(* Logix 5000 AddOnInstructionDefinition export POINT_ENC; software revision 30.00 *)

TYPE POINT :   // A point on an Edwards-curve represented in extended homogeneous coordinates
STRUCT
   X : DINT[22];
   Y : DINT[22];
   Z : DINT[22];
   T : DINT[22];
END_STRUCT
END_TYPE

ADD_ON_INSTRUCTION D_SHR   (* revision 1.0 20170524, vendor Kenneth A. Fischer *)
// DINT bit shift right of the 32-bit argument Inp_A by Inp_B bits with paddding by zeros on the right
// Revision note:
// Rev1.0: 20170524 - Initial Release
VAR_IN_OUT
   Inp_A : DINT; {required}   // 64-bit Integer to be right circular rotated
END_VAR
VAR_INPUT
   Inp_B : INT; {required}   // Number of bits to shift
END_VAR
VAR_IN_OUT
   Out : DINT; {required}   // Result
END_VAR
VAR
   BSR_Cntrl : CONTROL := (LEN := 32);
   ONS : BOOL;
   Source_Bit : BOOL;
   Wrk_InpA : DINT[2];
END_VAR

ROUTINE Logic   (* ladder *)
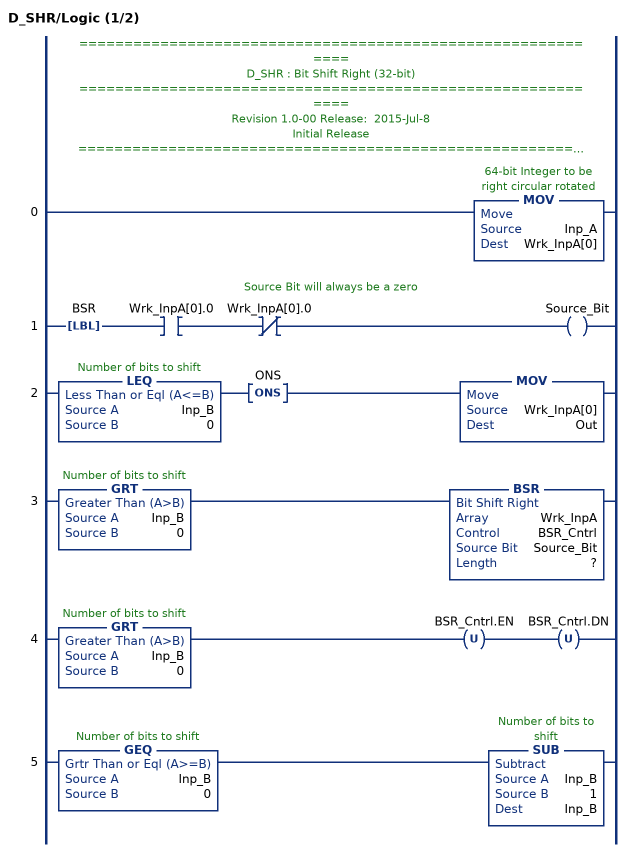
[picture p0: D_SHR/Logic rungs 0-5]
   // ============================================================
   // D_SHR : Bit Shift Right (32-bit)
   // ============================================================
   // Revision 1.0-00 Release:  2015-Jul-8
   // Initial Release
   // ============================================================
   // Performs a right bit shift of the 32-bit argument Inp_A by the
   // number of bits defined in the 16-bit argument Inp_B, with padding by zeros.
   0: MOV(Inp_A,Wrk_InpA[0]);
   // Source Bit will always be a zero
   1: LBL(BSR)XIC(Wrk_InpA[0].0)XIO(Wrk_InpA[0].0)OTE(Source_Bit);
   2: LEQ(Inp_B,0)ONS(ONS)MOV(Wrk_InpA[0],Out);
   3: GRT(Inp_B,0)BSR(Wrk_InpA,BSR_Cntrl,Source_Bit,?);
   4: GRT(Inp_B,0)OTU(BSR_Cntrl.EN)OTU(BSR_Cntrl.DN);
   5: GEQ(Inp_B,0)SUB(Inp_B,1,Inp_B);
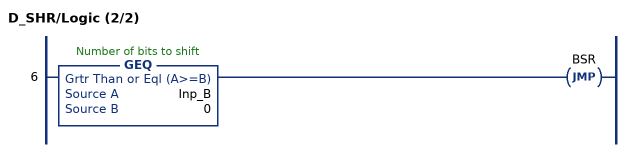
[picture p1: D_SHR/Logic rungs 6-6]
   6: GEQ(Inp_B,0)JMP(BSR);
END_ROUTINE
END_ADD_ON_INSTRUCTION

ADD_ON_INSTRUCTION B256_NRED   (* revision 1.0 20170916, vendor Kenneth A. Fischer *)
// Reduce 256-bit integer stored in 22 pieces by propagating carries
// Revision note:
// Rev1.0: 20170916 - Initial Release
VAR_IN_OUT
   Inp_C : DINT[22]; {required}
END_VAR
VAR
   D_SHR : D_SHR;
   temp : DINT;
   i : INT;
END_VAR

ROUTINE Logic   (* ladder *)
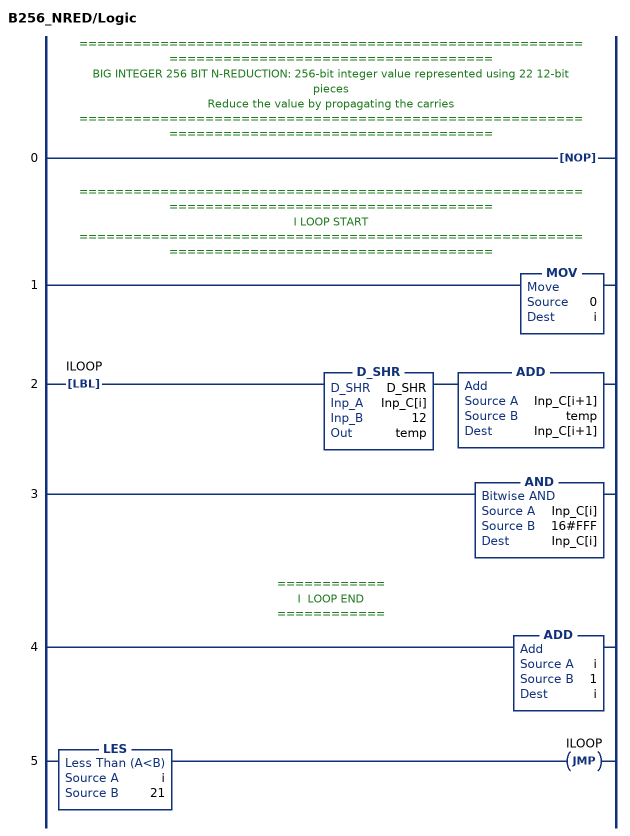
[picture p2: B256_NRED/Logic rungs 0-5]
   // ============================================================================================
   // BIG INTEGER 256 BIT N-REDUCTION: 256-bit integer value represented using 22 12-bit pieces
   // Reduce the value by propagating the carries
   // ============================================================================================
   0: NOP();
   // ============================================================================================
   // I LOOP START
   // ============================================================================================
   1: MOV(0,i);
   2: LBL(ILOOP)D_SHR(D_SHR,Inp_C[i],12,temp)ADD(Inp_C[i+1],temp,Inp_C[i+1]);
   3: AND(Inp_C[i],16#FFF,Inp_C[i]);
   // ============
   // I  LOOP END
   // ============
   4: ADD(i,1,i);
   5: LES(i,21)JMP(ILOOP);
END_ROUTINE
END_ADD_ON_INSTRUCTION

ADD_ON_INSTRUCTION B256_FRED   (* revision 1.0 20170916, vendor Kenneth A. Fischer *)
// fast_reduce:  reduce by propagating the carries starting at a particular offset and stoping once the carry becomes zero
// Revision note:
// Rev1.0: 20170916 - Initial Release
VAR_IN_OUT
   Inp_C : DINT[22]; {required}
END_VAR
VAR_INPUT
   Inp_offset : INT; {required}
END_VAR
VAR
   i : INT;
   carry : DINT;
   D_SHR : D_SHR;
END_VAR

ROUTINE Logic   (* ladder *)
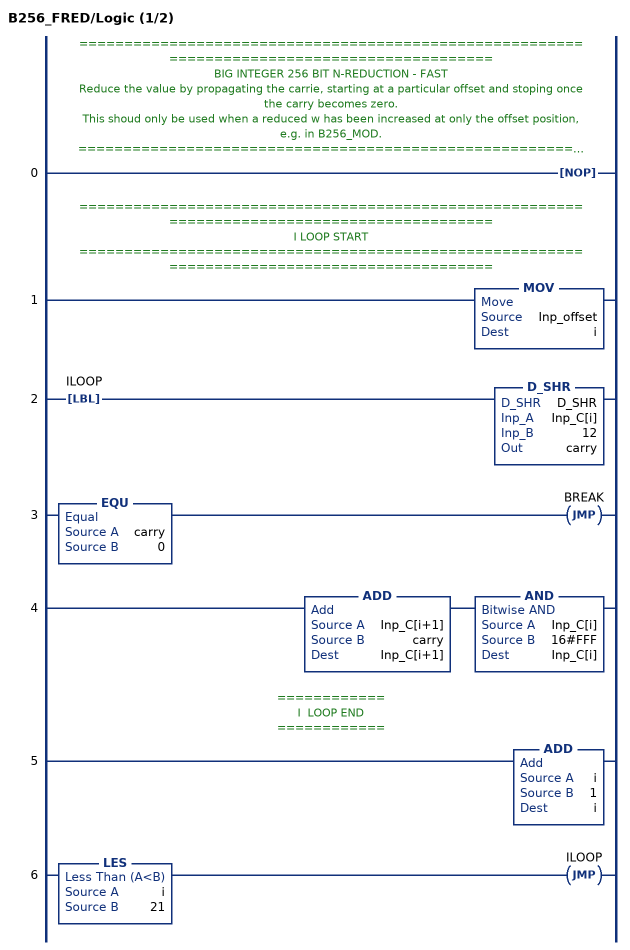
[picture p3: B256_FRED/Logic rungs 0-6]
   // ============================================================================================
   // BIG INTEGER 256 BIT N-REDUCTION - FAST
   // Reduce the value by propagating the carrie, starting at a particular offset and stoping once the carry becomes zero.
   // This shoud only be used when a reduced w has been increased at only the offset position, e.g. in B256_MOD.
   // ============================================================================================
   0: NOP();
   // ============================================================================================
   // I LOOP START
   // ============================================================================================
   1: MOV(Inp_offset,i);
   2: LBL(ILOOP)D_SHR(D_SHR,Inp_C[i],12,carry);
   3: EQU(carry,0)JMP(BREAK);
   4: ADD(Inp_C[i+1],carry,Inp_C[i+1])AND(Inp_C[i],16#FFF,Inp_C[i]);
   // ============
   // I  LOOP END
   // ============
   5: ADD(i,1,i);
   6: LES(i,21)JMP(ILOOP);
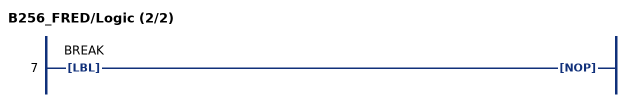
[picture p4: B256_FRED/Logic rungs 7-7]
   7: LBL(BREAK)NOP();
END_ROUTINE
END_ADD_ON_INSTRUCTION

ADD_ON_INSTRUCTION D_SHL   (* revision 1.0 20170524, vendor Kenneth A. Fischer *)
// DINT bit shift left of the 32-bit argument Inp_A by Inp_B bits with paddding by zeros on the right
// Revision note:
// Rev1.0: 20170524 - Initial Release
VAR_IN_OUT
   Inp_A : DINT; {required}   // 64-bit Integer to be right circular rotated
END_VAR
VAR_INPUT
   Inp_B : INT; {required}   // Number of bits to shift
END_VAR
VAR_IN_OUT
   Out : DINT; {required}   // Result
END_VAR
VAR
   Wrk_InpA : DINT[2];
   Source_Bit : BOOL;
   ONS : BOOL;
   BSL_Cntrl : CONTROL := (LEN := 32);
END_VAR

ROUTINE Logic   (* ladder *)
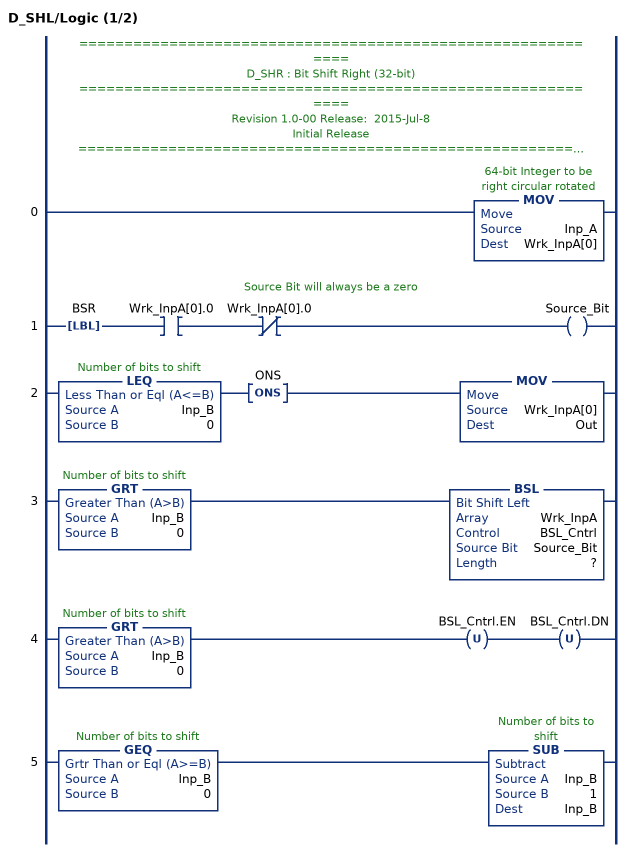
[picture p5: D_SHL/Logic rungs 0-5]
   // ============================================================
   // D_SHR : Bit Shift Right (32-bit)
   // ============================================================
   // Revision 1.0-00 Release:  2015-Jul-8
   // Initial Release
   // ============================================================
   // Performs a left bit shift of the 32-bit argument Inp_A by the
   // number of bits defined in the 16-bit argument Inp_B, with padding by zeros.
   0: MOV(Inp_A,Wrk_InpA[0]);
   // Source Bit will always be a zero
   1: LBL(BSR)XIC(Wrk_InpA[0].0)XIO(Wrk_InpA[0].0)OTE(Source_Bit);
   2: LEQ(Inp_B,0)ONS(ONS)MOV(Wrk_InpA[0],Out);
   3: GRT(Inp_B,0)BSL(Wrk_InpA,BSL_Cntrl,Source_Bit,?);
   4: GRT(Inp_B,0)OTU(BSL_Cntrl.EN)OTU(BSL_Cntrl.DN);
   5: GEQ(Inp_B,0)SUB(Inp_B,1,Inp_B);
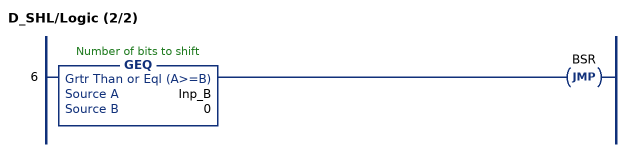
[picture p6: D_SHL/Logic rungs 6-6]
   6: GEQ(Inp_B,0)JMP(BSR);
END_ROUTINE
END_ADD_ON_INSTRUCTION

ADD_ON_INSTRUCTION B256_MOD   (* revision 1.0 20170916, vendor Kenneth A. Fischer *)
// c = d mod (2^255 - 19)
// Revision note:
// Rev1.0: 20170916 - Initial Release
VAR_IN_OUT
   Inp_D : DINT[43]; {required}
   Out_C : DINT[22]; {required}
END_VAR
VAR
   B256_NRED : B256_NRED;
   D_SHL : D_SHL;
   D_SHR : D_SHR;
   i : INT;
   t : DINT;
   temp : DINT;
   temp2 : DINT;
   B256_FRED : B256_FRED;
   offset : DINT;
END_VAR

ROUTINE Logic   (* ladder *)
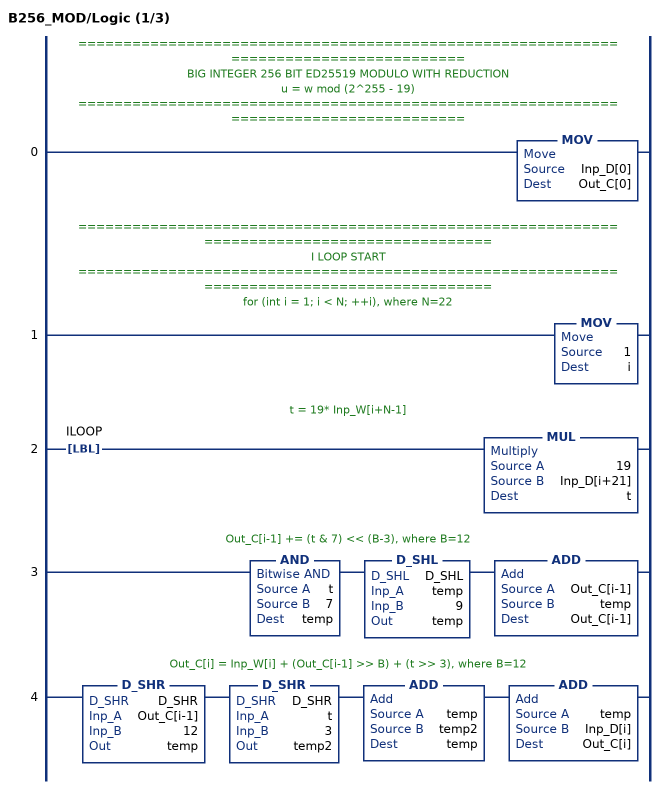
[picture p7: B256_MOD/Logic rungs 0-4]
   // ======================================================================================
   // BIG INTEGER 256 BIT ED25519 MODULO WITH REDUCTION
   //  u = w mod (2^255 - 19)
   // ======================================================================================
   0: MOV(Inp_D[0],Out_C[0]);
   // ============================================================================================
   // I LOOP START
   // ============================================================================================
   // for (int i = 1; i < N; ++i), where N=22
   1: MOV(1,i);
   // t = 19* Inp_W[i+N-1]
   2: LBL(ILOOP)MUL(19,Inp_D[i+21],t);
   // Out_C[i-1] += (t & 7) << (B-3), where B=12
   3: AND(t,7,temp)D_SHL(D_SHL,temp,9,temp)ADD(Out_C[i-1],temp,Out_C[i-1]);
   // Out_C[i] = Inp_W[i] + (Out_C[i-1] >> B) + (t >> 3), where B=12
   4: D_SHR(D_SHR,Out_C[i-1],12,temp)D_SHR(D_SHR,t,3,temp2)ADD(temp,temp2,temp)ADD(temp,Inp_D[i],Out_C[i]);
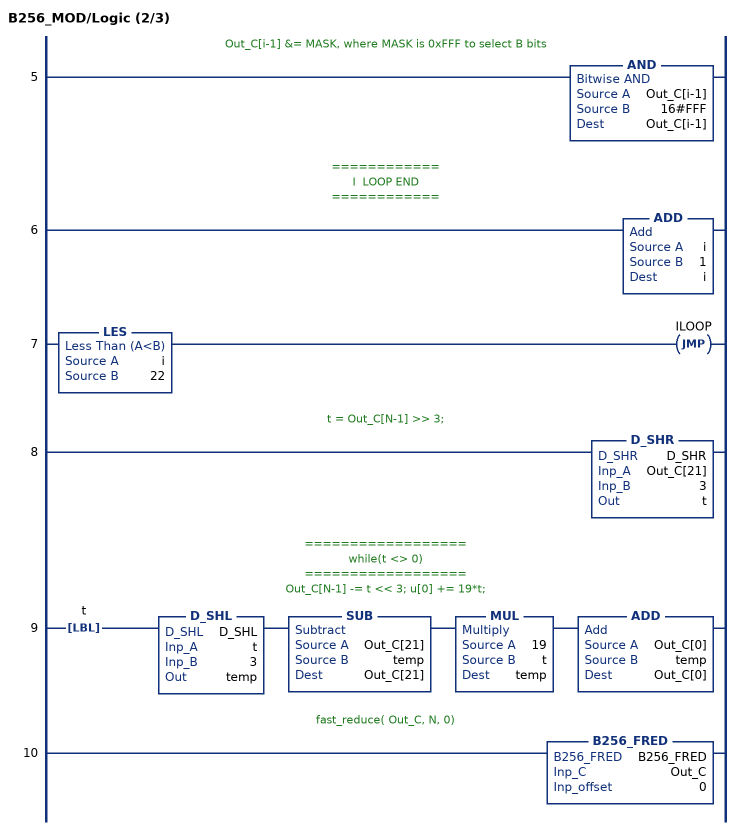
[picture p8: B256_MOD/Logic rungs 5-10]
   // Out_C[i-1] &= MASK, where MASK is 0xFFF to select B bits
   5: AND(Out_C[i-1],16#FFF,Out_C[i-1]);
   // ============
   // I  LOOP END
   // ============
   6: ADD(i,1,i);
   7: LES(i,22)JMP(ILOOP);
   // t = Out_C[N-1] >> 3;
   8: D_SHR(D_SHR,Out_C[21],3,t);
   // ==================
   // while(t <> 0)
   // ==================
   // Out_C[N-1] -= t << 3; u[0] += 19*t;
   9: LBL(t)D_SHL(D_SHL,t,3,temp)SUB(Out_C[21],temp,Out_C[21])MUL(19,t,temp)ADD(Out_C[0],temp,Out_C[0]);
   // fast_reduce( Out_C, N, 0)
   10: B256_FRED(B256_FRED,Out_C,0);
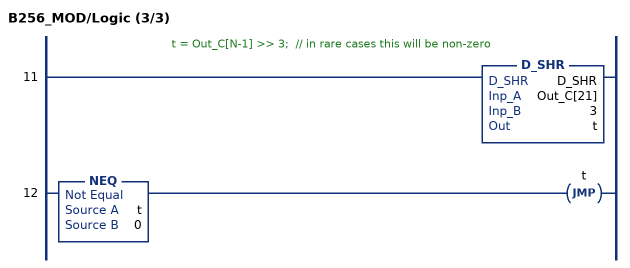
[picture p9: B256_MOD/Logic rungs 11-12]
   // t = Out_C[N-1] >> 3;  // in rare cases this will be non-zero
   11: D_SHR(D_SHR,Out_C[21],3,t);
   12: NEQ(t,0)JMP(t);
END_ROUTINE
END_ADD_ON_INSTRUCTION

ADD_ON_INSTRUCTION B256_NNRED   (* revision 1.0 20170916, vendor Kenneth A. Fischer *)
// Reduce 256-bit integer stored in 43 pieces by propagating carries
// Revision note:
// Rev1.0: 20170916 - Initial Release
VAR_IN_OUT
   Inp_D : DINT[43]; {required}
END_VAR
VAR
   temp : DINT;
   i : INT;
   D_SHR : D_SHR;
END_VAR

ROUTINE Logic   (* ladder *)
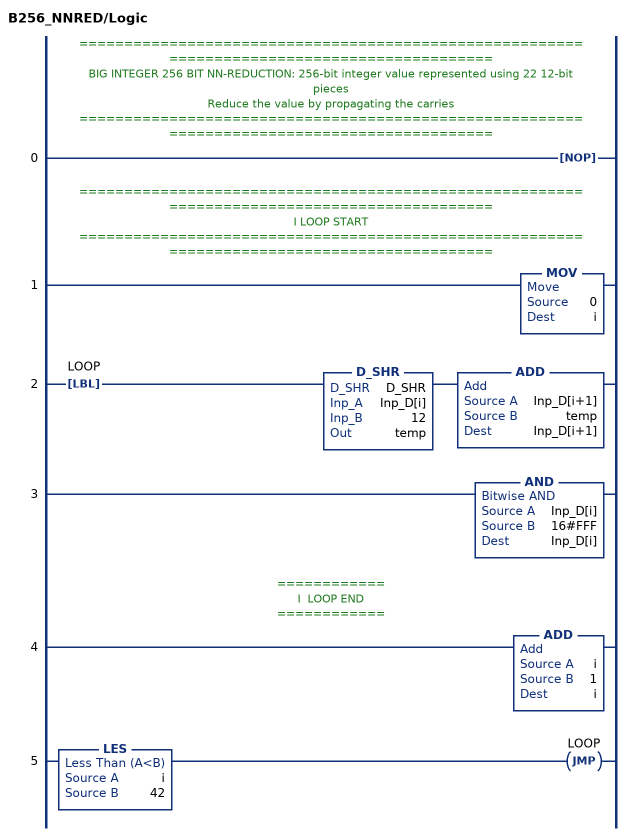
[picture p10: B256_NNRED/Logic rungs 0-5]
   // ============================================================================================
   // BIG INTEGER 256 BIT NN-REDUCTION: 256-bit integer value represented using 22 12-bit pieces
   // Reduce the value by propagating the carries
   // ============================================================================================
   0: NOP();
   // ============================================================================================
   // I LOOP START
   // ============================================================================================
   1: MOV(0,i);
   2: LBL(LOOP)D_SHR(D_SHR,Inp_D[i],12,temp)ADD(Inp_D[i+1],temp,Inp_D[i+1]);
   3: AND(Inp_D[i],16#FFF,Inp_D[i]);
   // ============
   // I  LOOP END
   // ============
   4: ADD(i,1,i);
   5: LES(i,42)JMP(LOOP);
END_ROUTINE
END_ADD_ON_INSTRUCTION

ADD_ON_INSTRUCTION B256_MUL   (* revision 1.0 20170916, vendor Kenneth A. Fischer *)
// c3 = c1*c2 with reduction and mod
// Revision note:
// Rev1.0: 20170916 - Initial Release
VAR_IN_OUT
   Temp_D : DINT[43]; {required}
   Inp_C1 : DINT[22]; {required}
   Inp_C2 : DINT[22]; {required}
   Out_C3 : DINT[22]; {required}
END_VAR
VAR
   B256_MOD : B256_MOD;
   B256_NNRED : B256_NNRED;
   i : INT;
   j : INT;
   mul_temp : DINT;
END_VAR

ROUTINE Logic   (* ladder *)
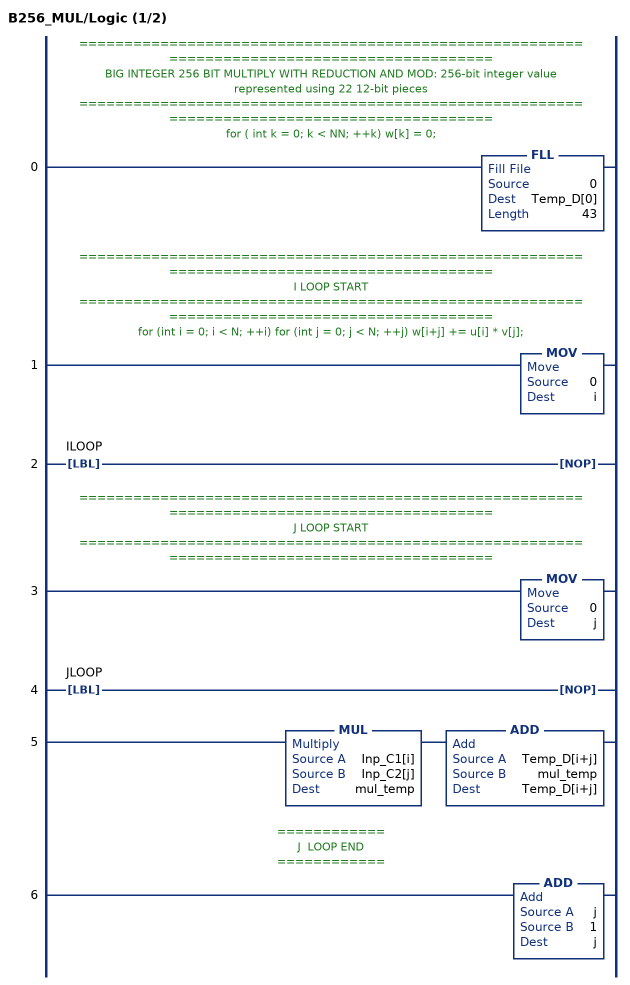
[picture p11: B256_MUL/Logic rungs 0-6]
   // ============================================================================================
   // BIG INTEGER 256 BIT MULTIPLY WITH REDUCTION AND MOD: 256-bit integer value represented using 22 12-bit pieces
   // ============================================================================================
   // for ( int k = 0; k < NN; ++k) w[k] = 0;
   0: FLL(0,Temp_D[0],43);
   // ============================================================================================
   // I LOOP START
   // ============================================================================================
   // for (int i = 0; i < N; ++i) for (int j = 0; j < N; ++j) w[i+j] += u[i] * v[j];
   1: MOV(0,i);
   2: LBL(ILOOP)NOP();
   // ============================================================================================
   // J LOOP START
   // ============================================================================================
   3: MOV(0,j);
   4: LBL(JLOOP)NOP();
   5: MUL(Inp_C1[i],Inp_C2[j],mul_temp)ADD(Temp_D[i+j],mul_temp,Temp_D[i+j]);
   // ============
   // J  LOOP END
   // ============
   6: ADD(j,1,j);
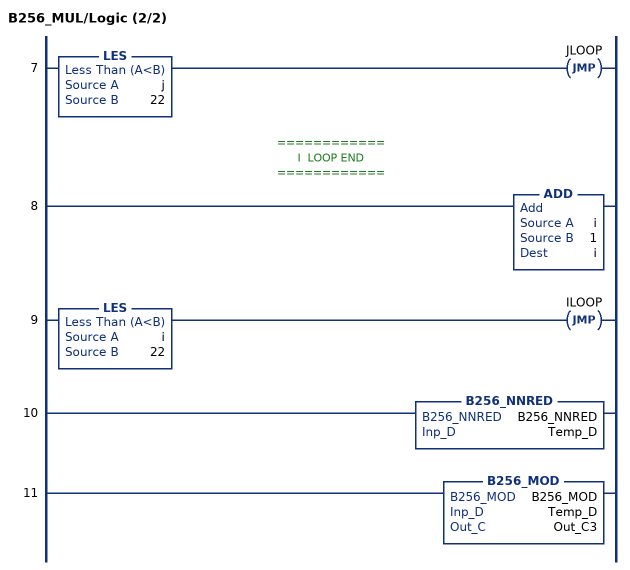
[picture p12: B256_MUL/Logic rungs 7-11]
   7: LES(j,22)JMP(JLOOP);
   // ============
   // I  LOOP END
   // ============
   8: ADD(i,1,i);
   9: LES(i,22)JMP(ILOOP);
   10: B256_NNRED(B256_NNRED,Temp_D);
   11: B256_MOD(B256_MOD,Temp_D,Out_C3);
END_ROUTINE
END_ADD_ON_INSTRUCTION

ADD_ON_INSTRUCTION B256_SQU   (* revision 1.0 20170916, vendor Kenneth A. Fischer *)
// c2 = c1*c1 with reduction and mod
// uses about half the number of multiplies compared to B256_MOD
// Revision note:
// Rev1.0: 20170916 - Initial Release
VAR_IN_OUT
   Temp_D : DINT[43]; {required}
   Inp_C1 : DINT[22]; {required}
   Out_C2 : DINT[22]; {required}
END_VAR
VAR
   B256_NNRED : B256_NNRED;
   i : INT;
   j : INT;
   z : INT;
   mul_temp : DINT;
   B256_MOD : B256_MOD;
   B256_NRED : B256_NRED;
   t : DINT;
END_VAR

ROUTINE Logic   (* ladder *)
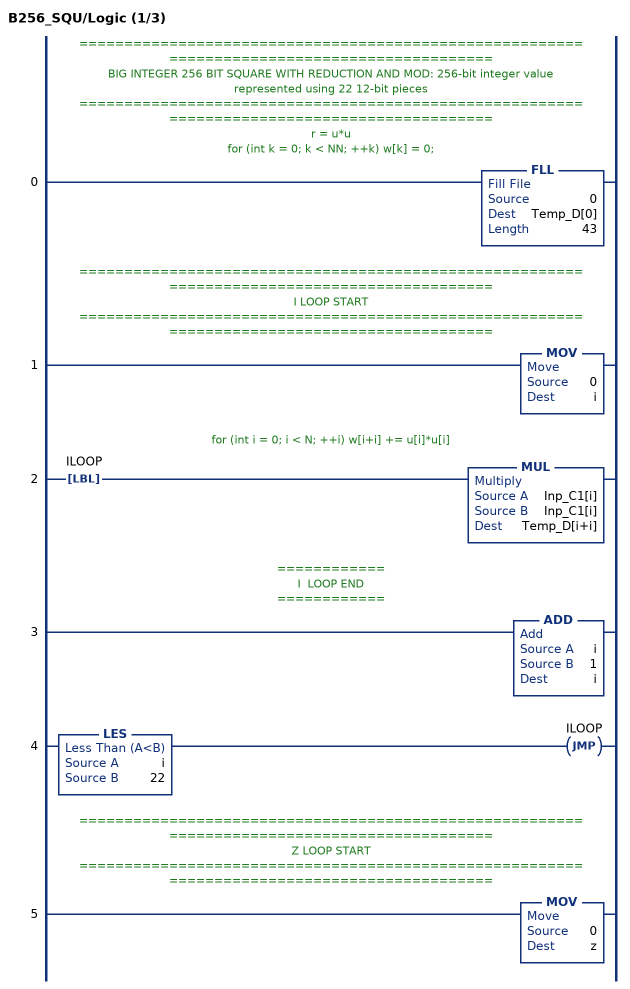
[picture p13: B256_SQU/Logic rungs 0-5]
   // ============================================================================================
   // BIG INTEGER 256 BIT SQUARE WITH REDUCTION AND MOD: 256-bit integer value represented using 22 12-bit pieces
   // ============================================================================================
   // r = u*u
   // for (int k = 0; k < NN; ++k) w[k] = 0;
   0: FLL(0,Temp_D[0],43);
   // ============================================================================================
   // I LOOP START
   // ============================================================================================
   1: MOV(0,i);
   // for (int i = 0; i < N; ++i) w[i+i] += u[i]*u[i]
   2: LBL(ILOOP)MUL(Inp_C1[i],Inp_C1[i],Temp_D[i+i]);
   // ============
   // I  LOOP END
   // ============
   3: ADD(i,1,i);
   4: LES(i,22)JMP(ILOOP);
   // ============================================================================================
   // Z LOOP START
   // ============================================================================================
   5: MOV(0,z);
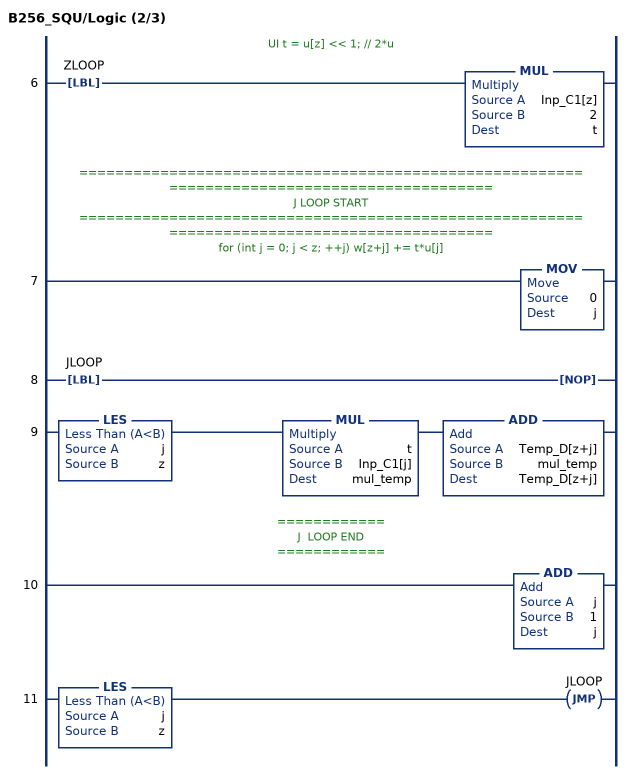
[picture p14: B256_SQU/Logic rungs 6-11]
   // UI t = u[z] << 1; // 2*u
   6: LBL(ZLOOP)MUL(Inp_C1[z],2,t);
   // ============================================================================================
   // J LOOP START
   // ============================================================================================
   // for (int j = 0; j < z; ++j) w[z+j] += t*u[j]
   7: MOV(0,j);
   8: LBL(JLOOP)NOP();
   9: LES(j,z)MUL(t,Inp_C1[j],mul_temp)ADD(Temp_D[z+j],mul_temp,Temp_D[z+j]);
   // ============
   // J  LOOP END
   // ============
   10: ADD(j,1,j);
   11: LES(j,z)JMP(JLOOP);
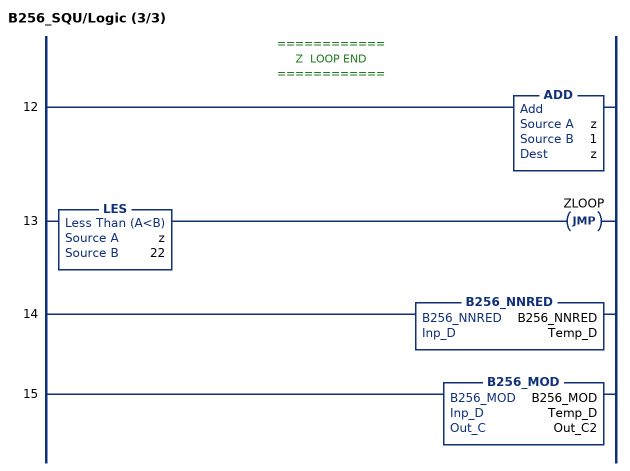
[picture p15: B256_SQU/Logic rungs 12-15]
   // ============
   // Z  LOOP END
   // ============
   12: ADD(z,1,z);
   13: LES(z,22)JMP(ZLOOP);
   14: B256_NNRED(B256_NNRED,Temp_D);
   15: B256_MOD(B256_MOD,Temp_D,Out_C2);
END_ROUTINE
END_ADD_ON_INSTRUCTION

ADD_ON_INSTRUCTION B256_ADJ   (* revision 1.0 20170916, vendor Kenneth A. Fischer *)
// if c >= m then subtract m
// Revision note:
// Rev1.0: 20170916 - Initial Release
VAR_IN_OUT
   Inp_C : DINT[22]; {required}
END_VAR
VAR
   i : INT;
   j : INT;
END_VAR

ROUTINE Logic   (* ladder *)
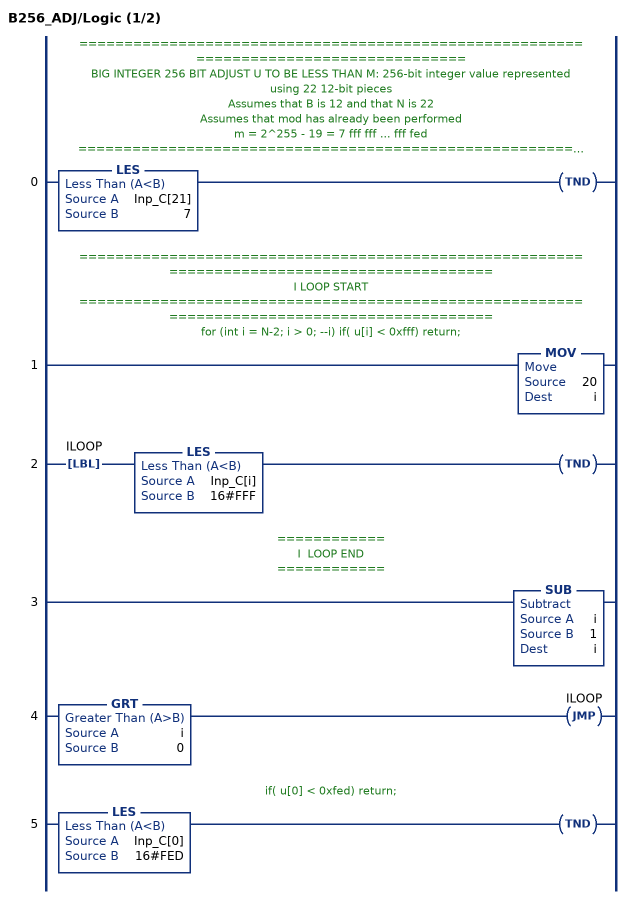
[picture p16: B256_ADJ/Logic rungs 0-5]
   // ======================================================================================
   // BIG INTEGER 256 BIT ADJUST U TO BE LESS THAN M: 256-bit integer value represented using 22 12-bit pieces
   // Assumes that B is 12 and that N is 22
   // Assumes that mod has already been performed
   // m = 2^255 - 19 = 7 fff fff ... fff fed
   // ======================================================================================
   // if (u[n-1] < 7) return;
   0: LES(Inp_C[21],7)TND();
   // ============================================================================================
   // I LOOP START
   // ============================================================================================
   // for (int i = N-2; i > 0; --i) if( u[i] < 0xfff) return;
   1: MOV(20,i);
   2: LBL(ILOOP)LES(Inp_C[i],16#FFF)TND();
   // ============
   // I  LOOP END
   // ============
   3: SUB(i,1,i);
   4: GRT(i,0)JMP(ILOOP);
   // if( u[0] < 0xfed) return;
   5: LES(Inp_C[0],16#FED)TND();
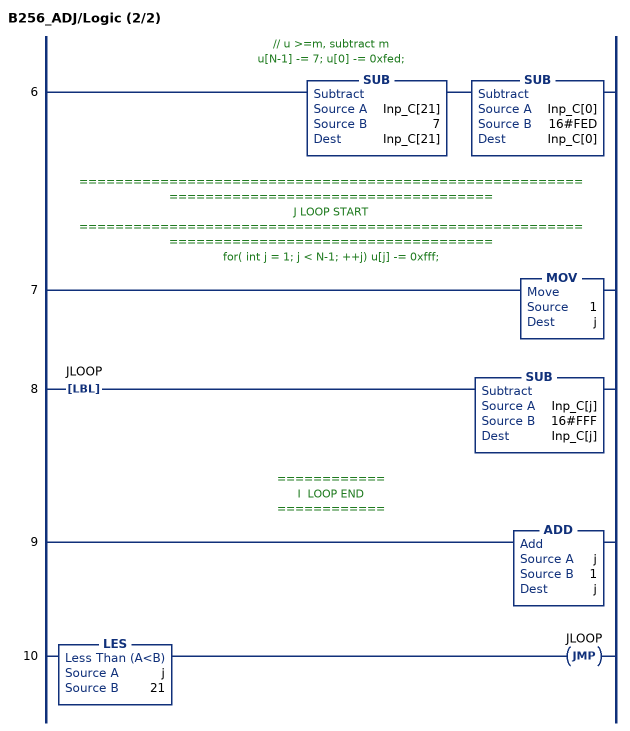
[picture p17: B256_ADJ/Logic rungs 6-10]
   // // u >=m, subtract m
   // u[N-1] -= 7; u[0] -= 0xfed;
   6: SUB(Inp_C[21],7,Inp_C[21])SUB(Inp_C[0],16#FED,Inp_C[0]);
   // ============================================================================================
   // J LOOP START
   // ============================================================================================
   // for( int j = 1; j < N-1; ++j) u[j] -= 0xfff;
   7: MOV(1,j);
   8: LBL(JLOOP)SUB(Inp_C[j],16#FFF,Inp_C[j]);
   // ============
   // I  LOOP END
   // ============
   9: ADD(j,1,j);
   10: LES(j,21)JMP(JLOOP);
END_ROUTINE
END_ADD_ON_INSTRUCTION
